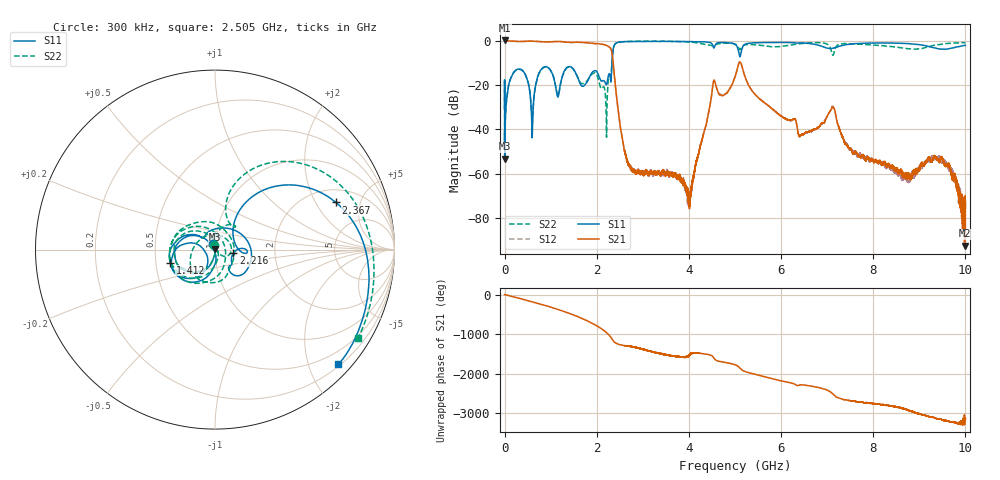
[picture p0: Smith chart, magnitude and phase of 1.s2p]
!Keysight Technologies,N5232A,MY52221221,A.10.65.11
!Date: Thursday, March 30, 2023 15:33:23
!Correction: S11(Full 2 Port(1,4))
!S41(Full 2 Port(1,4))
!S14(Full 2 Port(1,4))
!S44(Full 2 Port(1,4))
!S2P File: Measurements: S11, S41, S14, S44:
# Hz S  RI  R 50
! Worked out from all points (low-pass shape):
!   16001 points, 300 kHz to 10 GHz, reference 50 ohm
!   highest |S21| = 0.10 dB at 300 kHz (marker M1); lowest = -92.5 dB at 9.983 GHz (marker M2)
!   |S21| within 3 dB of the highest: start of sweep to 2.276 GHz
!   lowest |S11| = -53.2 dB at 2.8 MHz (marker M3), VSWR 1.00, Z = 50.1 + j0.166 ohm
!   |S11| at or under -10 dB: start of sweep to 2.33 GHz
!   |S22| runs from -53.9 to -0.2 dB; largest |S21 - S12| = 0.013
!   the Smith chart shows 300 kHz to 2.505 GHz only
!   S11 on the Smith chart (normalised r, x): 300 kHz: 0.98, +0.06; 1.412 GHz: 0.60, -0.09; 2.216 GHz: 1.23, -0.05; 2.367 GHz: 2.72, +2.99; 2.505 GHz: 0.23, -2.53
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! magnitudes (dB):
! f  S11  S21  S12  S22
! 300 kHz  -30.4  0.1  0.1  -30.9
! 2.8 MHz  -53.2  0.0  0.0  -53.9
! 250.3 MHz  -13.2  -0.3  -0.3  -13.1
! 599 MHz  -43.8  -0.2  -0.2  -37.1
! 804.7 MHz  -12.7  -0.5  -0.5  -12.9
! 1.155 GHz  -25.4  -0.4  -0.4  -24.9
! 1.412 GHz  -11.7  -0.7  -0.7  -11.8
! 1.667 GHz  -20.3  -0.7  -0.7  -19.3
! 2.216 GHz  -19.6  -2.1  -2.1  -35.9
! 2.367 GHz  -2.8  -12.4  -12.6  -2.9
! 2.505 GHz  -0.5  -38.3  -37.7  -0.6
! 2.746 GHz  -0.4  -57.9  -57.3  -0.3
! 3.334 GHz  -0.3  -59.7  -60.2  -0.2
! 4.011 GHz  -0.4  -75.2  -73.6  -0.7
! 4.533 GHz  -3.0  -18.4  -18.5  -2.4
! 5 GHz  -1.6  -16.4  -16.1  -1.5
! 6.667 GHz  -1.4  -40.6  -40.9  -0.9
! 7.122 GHz  -3.4  -30.0  -29.5  -6.5
! 8.334 GHz  -1.1  -55.8  -56.1  -2.5
! 9.491 GHz  -3.8  -52.8  -54.5  -1.5
! 9.983 GHz  -2.1  -92.5  -82.2  -0.9
! 10 GHz  -2.1  -86.8  -75.9  -0.9
